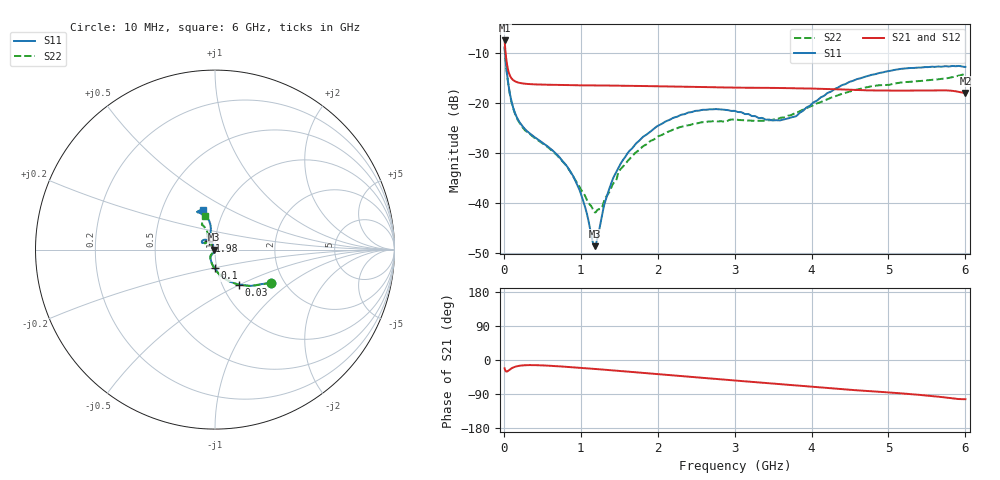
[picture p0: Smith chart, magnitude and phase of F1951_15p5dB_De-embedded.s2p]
! Integrated Device Technology
! Corporate Headquarters
! 6024 Silver Creek Valley Road
! San Jose, CA 95138  USA
! Phone:  1-408-284-8200
! Toll Free:  1-800-223-1366
! Webpage:  http://www.idt.com/
! Timing and RF Division
! 515 Groton Road, Suite 102
! Westford, MA 01886-6024
! Device:  F1951
! Description: 6-bit 0.5 dB Digital Step Attenuator
! Frequency:  100.0 -  4000.00 MHz
! Package:  4x4 mm Thin QFN Plastic Package: 24 pin
! Ports:  2 RF, 6 DC
!  Pin  1  = NC
!  Pin  2  = RF1  =  Port 1
!  Pin  3  = GND
!  Pin  4  = NC
!  Pin  5  = Serial Data Out (SDO)
!  Pin  6  = NC
!  Pin  7  = Reset Bar ( RSTb)
!  Pin  8  = Clock (CLK)
!  Pin  9  = Chip Select Bar (CSb)
!  Pin 10  = NC
!  Pin 11  = Serial Data In (SDI)
!  Pin 12  = NC
!  Pin 13  = NC
!  Pin 14  = VDD
!  Pin 15  = NC
!  Pin 16  = GND
!  Pin 17  = RF2  =  Port 2
!  Pin 18  = NC
!  Pin 19  = GND
!  Pin 20  = GND
!  Pin 21  = GND
!  Pin 22  = GND
!  Pin 23  = GND
!  Pin 24  = GND
! State:  31
! Atten State:  15.5 dB
! Voltage:  +3.30 Volts
! Current:  0.483 mA
! Data:  The device was measured on a F195X evaluation board which has
!  individual transmission lines to the RF pins.  Data was collected
!  de-embedded using a Automatic Fixture Removal [AFR] (Keysight Technologies).
!  The reference plane is the edge of the package pin.
! Misc:  Lot Code  1225BCA
!  Action Tracker AT0399
! Date Measured:  2018-09-13
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# GHz S dB R 50
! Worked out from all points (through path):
!   600 points, 10 MHz to 6 GHz, reference 50 ohm
!   highest |S21| = -7.47 dB at 10 MHz (marker M1); lowest = -18.0 dB at 6 GHz (marker M2)
!   group delay of S21, straight-line fit = 43.6 ps
!   lowest |S11| = -48.7 dB at 1.18 GHz (marker M3), VSWR 1.01, Z = 49.6 + j0.0179 ohm
!   |S11| at or under -10 dB: 15.66 MHz to end of sweep
!   |S22| runs from -41.9 to -8.8 dB; largest |S21 - S12| = 0.00031
!   S11 on the Smith chart (normalised r, x): 10 MHz: 1.71, -0.72; 30 MHz: 1.19, -0.49; 100 MHz: 0.97, -0.20; 1.98 GHz: 0.94, +0.09; 6 GHz: 0.80, +0.37
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0.01  -8.82 -30.5  -7.47 -22.0  -7.47 -22.0  -8.84 -31.0
0.03  -12.55 -55.8  -10.97 -30.4  -10.97 -30.4  -12.66 -56.8
0.06  -16.37 -76.3  -13.66 -27.9  -13.67 -27.9  -16.53 -77.5
0.1  -19.71 -91.5  -15.06 -22.0  -15.07 -22.0  -19.84 -93.1
0.25  -24.80 -115.3  -16.10 -14.1  -16.10 -14.1  -25.00 -117.8
0.72  -30.80 -118.8  -16.38 -16.7  -16.38 -16.7  -30.98 -127.6
0.89  -34.35 -116.7  -16.43 -19.2  -16.43 -19.2  -34.41 -128.7
1.01  -38.57 -117.9  -16.46 -20.9  -16.46 -20.9  -37.54 -133.2
1.18  -48.69 177.2  -16.48 -23.5  -16.49 -23.5  -41.88 -169.8
1.26  -43.76 123.0  -16.49 -24.8  -16.49 -24.8  -41.23 163.4
1.34  -38.68 111.5  -16.50 -26.2  -16.51 -26.2  -38.56 144.5
1.5  -32.71 108.7  -16.55 -28.7  -16.55 -28.7  -33.57 129.9
1.72  -28.09 114.1  -16.58 -32.5  -16.58 -32.5  -29.86 126.4
1.98  -24.79 122.6  -16.64 -37.0  -16.64 -37.0  -26.97 130.3
2.01  -24.52 124.0  -16.65 -37.5  -16.65 -37.5  -26.66 131.4
2.49  -21.58 139.6  -16.78 -45.7  -16.78 -45.7  -24.11 141.7
3.01  -21.62 151.4  -16.91 -54.3  -16.92 -54.3  -23.31 146.5
3.59  -23.49 129.9  -16.99 -63.9  -17.00 -63.9  -23.00 127.8
4.01  -20.09 104.2  -17.11 -70.9  -17.11 -70.9  -20.55 115.3
4.49  -15.79 101.4  -17.35 -78.5  -17.35 -78.5  -17.73 114.2
5.01  -13.61 110.1  -17.53 -85.7  -17.53 -85.6  -16.36 117.4
6  -12.76 107.5  -17.98 -103.4  -17.98 -103.4  -14.15 105.9
